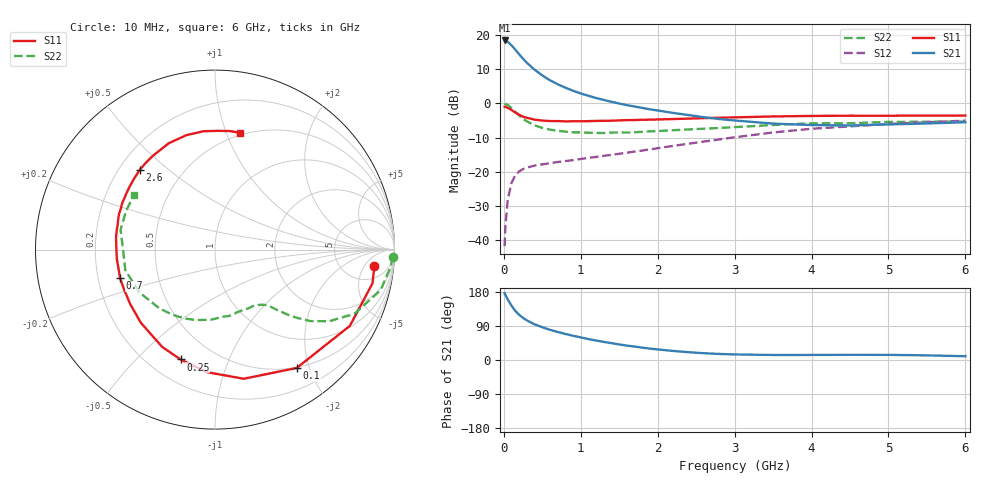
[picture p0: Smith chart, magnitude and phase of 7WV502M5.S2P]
! Infineon Technologies  Discrete & RF Semiconductors
! BFS17W
! Si NPN RF Bipolar Junction Transistor in SOT323
! VCE = 0.5 V  IC = 2.5 mA
! Common Emitter S-Parameters:  August  1999
# GHz  S  MA  R  50
!  f  S11  S21  S12  S22
! GHz  MAG  ANG  MAG  ANG  MAG  ANG  MAG  ANG
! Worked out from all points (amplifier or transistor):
!   36 points, 10 MHz to 6 GHz, reference 50 ohm
!   highest |S21| = 18.4 dB at 10 MHz (marker M1)
!   |S21| within 3 dB of that: start of sweep to 160.6 MHz
!   unconditionally stable (mu >= 1): 639.8 MHz to end of sweep
!   at 250 MHz: K = 0.45, MSG = 16.1 dB, |S12| = -19.2 dB
!   at 1.4 GHz: K = 1.46, MAG = 3.7 dB, |S12| = -15.0 dB
!   at 6 GHz: K = 1.15, MAG = -2.6 dB, |S12| = -5.0 dB
!   S11 on the Smith chart (normalised r, x): 10 MHz: 10, -9; 100 MHz: 0.49, -1.80; 250 MHz: 0.33, -0.68; 700 MHz: 0.29, -0.13; 2.6 GHz: 0.28, +0.40; 6 GHz: 0.48, +1.12
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0.01  0.8927 -6.0  8.341 176.6  0.0082 84.2  0.9926 -2.4
0.02  0.8973 -12.1  8.292 172.0  0.0157 80.2  0.983 -5.7
0.05  0.8632 -29.5  8.001 159.9  0.039 74.4  0.9501 -13.7
0.1  0.8013 -55.4  7.086 143.2  0.0689 60.8  0.8555 -24.7
0.15  0.737 -77.5  6.102 129.3  0.0893 50.4  0.7509 -32.1
0.2  0.6841 -93.9  5.224 119.2  0.1019 44.5  0.6651 -36.8
0.25  0.6413 -107.4  4.5 111.1  0.1098 39.7  0.5964 -39.7
0.3  0.6172 -118.4  3.931 104.6  0.1155 36.9  0.5478 -41.7
0.4  0.5806 -135.2  3.116 94.2  0.1235 33.7  0.4789 -44.3
0.5  0.5619 -147.0  2.57 86.4  0.1287 32.7  0.4405 -45.9
0.6  0.5532 -156.0  2.182 79.7  0.1339 32.8  0.4147 -47.9
0.7  0.5525 -163.3  1.911 74.0  0.1395 33.4  0.3988 -50.4
0.9  0.5493 -174.7  1.534 64.0  0.1485 35.0  0.3789 -56.3
1.1  0.5519 176.1  1.294 55.2  0.1602 37.0  0.3734 -63.0
1.3  0.5583 168.4  1.126 47.7  0.1717 39.0  0.3702 -70.7
1.6  0.5711 159.2  0.945 38.0  0.1903 41.7  0.3762 -82.0
2.2  0.5918 143.3  0.728 23.9  0.2395 45.3  0.4064 -104.9
2.6  0.6105 133.5  0.63 17.9  0.2772 45.6  0.4275 -119.9
3.5  0.6462 113.5  0.508 13.2  0.3766 41.3  0.4841 -150.5
4.5  0.6626 95.5  0.476 13.7  0.4621 31.1  0.5137 178.8
5.5  0.6658 82.8  0.51 12.2  0.5317 21.6  0.5405 156.1
6  0.6652 78.0  0.532 9.9  0.5609 16.9  0.5436 146.0
